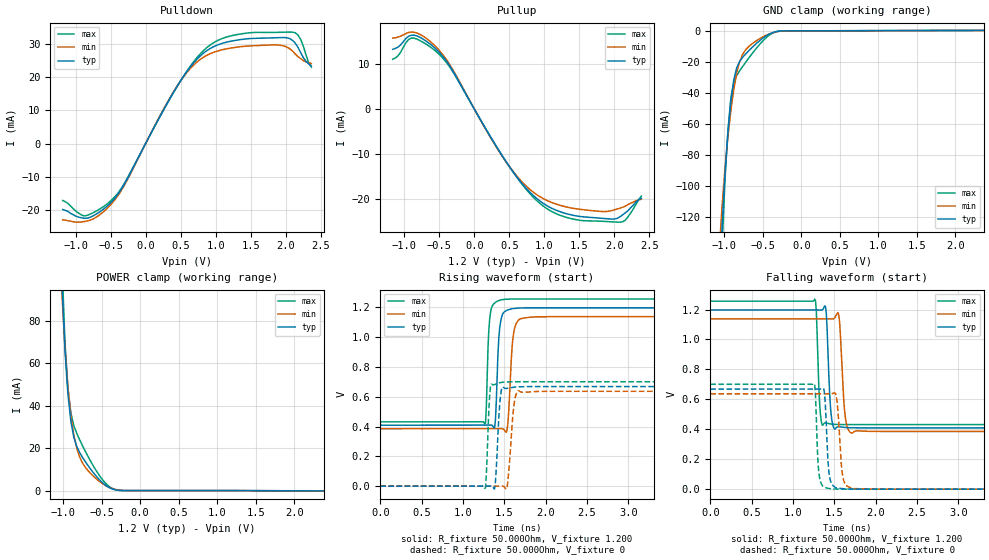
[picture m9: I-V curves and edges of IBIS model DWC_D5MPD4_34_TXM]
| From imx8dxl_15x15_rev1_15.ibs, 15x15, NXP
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[Model] DWC_D5MPD4_34_TXM
Model_type   I/O
Polarity   Non-Inverting
Enable   Active-High
C_comp   1.452pF   1.359pF   1.567pF
C_comp_pullup   326.913fF   306.621fF   352.138fF
C_comp_pulldown 1.100pF   1.017pF   1.196pF
Vinh = 910.000mV
Vinl = 724.000mV
Vmeas = 817.000mV
Vref = 817.000mV
Rref = 50Ohms
Cref = 0pF
[Model Spec]
Vinh   910.000mV   869.000mV   951.000mV
Vinl   724.000mV   683.000mV   765.000mV
Vmeas   817.000mV   776.000mV   858.000mV
Vref   817.000mV   776.000mV   858.000mV
D_overshoot_ampl_h 0.4 NA   NA
D_overshoot_ampl_l 0.4 NA   NA
D_overshoot_area_l 60.000p NA   NA
D_overshoot_area_h 60.000p NA   NA
[Receiver Thresholds]
Vcross_low = 697.000mV
Vcross_high = 937.000mV
Vdiff_ac = 136.000mV
Vdiff_dc = 136.000mV
Tdiffslew_ac = 10.000ns
[Temperature Range]   25.000   125.000   -40.000
[Voltage Range]   1.200V   1.140V   1.260V
[GND Clamp Reference]   0.00V   0.00V   0.00V
[C Comp Corner]
| variable   typ   min   max
C_comp 1.452pF   1.567pF   1.359pF
C_comp_pullup 326.913fF   352.138fF   306.621fF
C_comp_pulldown 1.100pF   1.196pF   1.017pF
[Pulldown Reference]   0.00V   0.00V   0.00V
[POWER Clamp Reference]   1.200V   1.140V   1.260V
[Pullup Reference]   1.200V   1.140V   1.260V
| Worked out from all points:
|   slope of the pulldown table from 0 to 0.18 V, typ, clamps not added: 25.1 ohm
|   slope of the pullup table from 0 to 0.18 V, typ, clamps not added: 37.1 ohm
|   GND clamp passes 1 mA (typ) near -0.36 V on its own axis
|   POWER clamp passes 1 mA (typ) near -0.38 V on its own axis
|   rising waveform, R_fixture 50.000Ohm, V_fixture 1.200: 20-80 % time 37.7ps typ, 46.6ps min, 32.9ps max; typ from 0.409 V to 1.2 V
|   rising waveform, R_fixture 50.000Ohm, V_fixture 0: 20-80 % time 38ps typ, 51.8ps min, 30.7ps max; typ from 0 V to 0.668 V
|   falling waveform, R_fixture 50.000Ohm, V_fixture 1.200: 20-80 % time 36.7ps typ, 44.9ps min, 31.5ps max; typ from 1.2 V to 0.409 V
|   falling waveform, R_fixture 50.000Ohm, V_fixture 0: 20-80 % time 37.4ps typ, 46.4ps min, 31.2ps max; typ from 0.668 V to 0 V
[GND Clamp]
-1.184V   -348.5mA   -259.9mA   -439.9mA
-1.069V   -169.5mA   -142.4mA   -196.8mA
-1.031V   -126.4mA   -112.9mA   -139.4mA
-954.5mV  -65.34mA   -67.95mA   -63.85mA
-916.4mV  -45.2mA    -51.17mA   -43.27mA
-878.2mV  -31.45mA   -37.57mA   -33.15mA
-840mV    -23.64mA   -27.11mA   -28.67mA
-763.6mV  -17.03mA   -15.11mA   -22.94mA
-610.9mV  -9.282mA   -7.243mA   -12.78mA
-420mV    -2.151mA   -2.011mA   -2.842mA
-267.3mV  -90.01uA   -209.5uA   -60.56uA
2.367V    273.5uA    222.3uA    340.9uA
[Power Clamp]
-1.167V   319.3mA    247.1mA    390.6mA
-1.015V   97.56mA    92.13mA    106.5mA
-976.4mV  66.14mA    67.19mA    69.94mA
-938.2mV  45.51mA    48.6mA     48.18mA
-900mV    32.73mA    35.4mA     36.58mA
-861.8mV  25.19mA    26.24mA    30.62mA
-823.6mV  20.79mA    20mA       26.94mA
-747.3mV  15.56mA    12.93mA    21.03mA
-518.2mV  4.741mA    4.028mA    6.547mA
-403.6mV  1.468mA    1.527mA    1.973mA
-250.9mV  45.67uA    138.5uA    40.26uA
2.384V    -136.7uA   -117uA     -161.8uA
[Pulldown]
-1.184V   -19.8mA    -22.9mA    -17.1mA
-878.2mV  -22.44mA   -23.43mA   -21.73mA
-458.2mV  -16.9mA    -17.39mA   -16.4mA
-305.5mV  -12.28mA   -12.62mA   -12.05mA
496.4mV   18.72mA    18.68mA    18.73mA
725.5mV   25.13mA    24.32mA    25.6mA
992.7mV   29.29mA    27.54mA    30.54mA
1.336V    31.15mA    29.02mA    32.82mA
1.871V    31.77mA    29.61mA    33.38mA
2.138V    30.14mA    26.89mA    33.25mA
2.215V    27.29mA    25.5mA     31.27mA
2.367V    23.3mA     24mA       22.9mA
[Pullup]
-1.167V   13.3mA     15.8mA     11.09mA
-900mV    16.42mA    17.12mA    15.79mA
-518.2mV  12.88mA    13.33mA    12.4mA
-327.3mV  9.001mA    9.273mA    8.784mA
207.3mV   -5.564mA   -5.684mA   -5.511mA
512.7mV   -13.03mA   -13mA      -13.06mA
780mV     -18.22mA   -17.64mA   -18.53mA
1.085V    -21.84mA   -20.59mA   -22.55mA
1.544V    -23.88mA   -22.29mA   -24.73mA
2.002V    -24.37mA   -22.33mA   -25.04mA
2.116V    -23.46mA   -21.78mA   -25mA
2.384V    -19.8mA    -19.99mA   -19.3mA
[Ramp]
R_load=50.000Ohm
dV/dt_r   436.860mV/38.500ps  416.789mV/49.500ps  457.530mV/32.000ps
dV/dt_f   436.860mV/37.500ps  416.789mV/46.000ps  457.530mV/31.500ps
[Rising waveform]
R_fixture=50.000Ohm
V_fixture=1.200
V_fixture_min=1.140
V_fixture_max=1.260
0s        409.4mV    385.5mV    431.9mV
1.263ns   409.4mV    385.5mV    417.3mV
1.323ns   410.3mV    385.5mV    1.119V
1.383ns   390.4mV    385.4mV    1.229V
1.434ns   995.1mV    386.3mV    1.246V
1.484ns   1.159V     383.7mV    1.253V
1.534ns   1.181V     377.2mV    1.255V
1.624ns   1.193V     1.058V     1.256V
1.764ns   1.197V     1.131V     1.256V
10ns      1.197V     1.138V     1.256V
[Rising waveform]
R_fixture=50.000Ohm
V_fixture=0
0s        142.6nV    3.545uV    17.79nV
1.273ns   -36.31uV   325.6nV    -10.51mV
1.323ns   664.5uV    15.34uV    605.5mV
1.383ns   -18.76mV   -88.75uV   682.1mV
1.444ns   544.8mV    921.7uV    694.1mV
1.474ns   662.8mV    1.283mV    697.2mV
1.534ns   656.5mV    -7.775mV   700mV
1.614ns   664.3mV    529.6mV    700.9mV
1.664ns   666.7mV    640.6mV    701.1mV
10ns      668.5mV    637mV      700.8mV
[Falling waveform]
R_fixture=50.000Ohm
V_fixture=1.200
V_fixture_min=1.140
V_fixture_max=1.260
0s        1.197V     1.138V     1.256V
1.263ns   1.197V     1.138V     1.27V
1.353ns   1.197V     1.138V     428.1mV
1.403ns   1.18V      1.138V     441.6mV
1.454ns   548.6mV    1.137V     435.7mV
1.504ns   401.2mV    1.144V     433mV
1.554ns   417.1mV    1.167V     432mV
1.624ns   412.5mV    528.2mV    431.7mV
1.714ns   410mV      374.3mV    431.6mV
10ns      409.4mV    385.5mV    431.8mV
[Falling waveform]
R_fixture=50.000Ohm
V_fixture=0
0s        668.5mV    637mV      700.7mV
1.263ns   668.5mV    637mV      701.3mV
1.323ns   668.1mV    637mV      72.68mV
1.383ns   634.1mV    637mV      12.73mV
1.423ns   194.1mV    636.7mV    5.937mV
1.454ns   56.16mV    636.7mV    3.054mV
1.524ns   8.984mV    623.1mV    664.9uV
1.614ns   2.497mV    57.29mV    103.6uV
1.734ns   324.4uV    4.305mV    24.27uV
10ns      339.8nV    3.765uV    258.8nV
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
